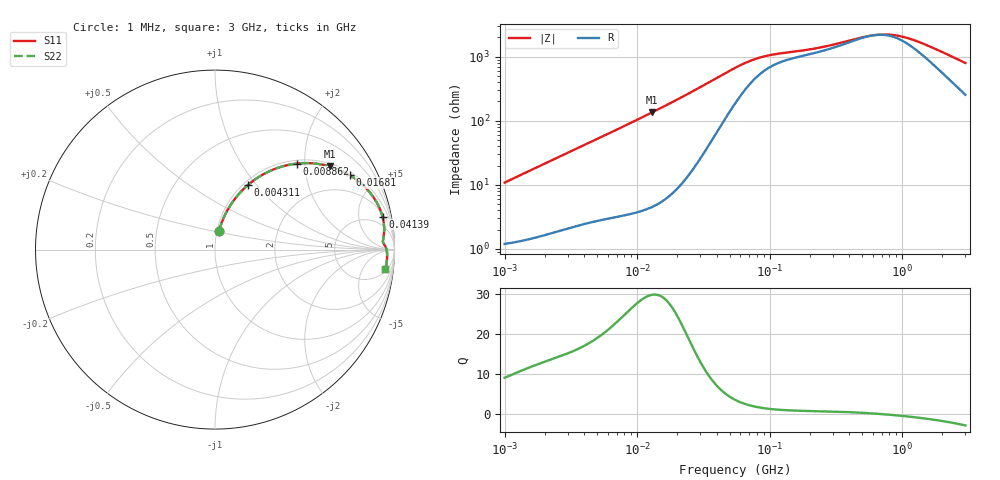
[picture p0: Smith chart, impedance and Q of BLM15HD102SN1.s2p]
! BLM15HD102SN1
# Hz S RI R 50
!Freq.(Hz) S11(Real) S11(Imag) S21(Real) S21(Imag) S12(Real) S12(Imag) S22(Real) S22(Imag)
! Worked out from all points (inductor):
!   401 points, 1 MHz to 3 GHz, reference 50 ohm
!   read as one part in series: L = 1.71 uH near 1.041 MHz
!   highest Q = 29.8 at 12.96 MHz (marker M1), where L = 1.65 uH
!   self-resonance near 622.8 MHz
!   S11 on the Smith chart (normalised r, x): 1 MHz: 1.02, +0.22; 4.311 MHz: 1.05, +0.90; 8.862 MHz: 1.07, +1.83; 16.81 MHz: 1.13, +3.54; 41.39 MHz: 2.49, +9.61; 3 GHz: 6, -15
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1000000  0.0229 0.1041  0.9771 -0.1041  0.9771 -0.1041  0.0229 0.1041
2139570  0.0637 0.2096  0.9363 -0.2096  0.9363 -0.2096  0.0637 0.2096
2888807  0.1003 0.2687  0.8997 -0.2687  0.8997 -0.2687  0.1003 0.2687
3823119  0.1526 0.3309  0.8474 -0.3309  0.8474 -0.3309  0.1526 0.3309
4310966  0.1819 0.3584  0.8181 -0.3584  0.8181 -0.3584  0.1819 0.3584
6058321  0.2914 0.4313  0.7086 -0.4313  0.7086 -0.4313  0.2914 0.4313
8861669  0.4577 0.4794  0.5423 -0.4794  0.5423 -0.4794  0.4577 0.4794
1.29622e7  0.6405 0.4634  0.3595 -0.4634  0.3595 -0.4634  0.6405 0.4634
1.461624e7  0.6939 0.4443  0.3061 -0.4443  0.3061 -0.4443  0.6939 0.4443
1.681455e7  0.7503 0.4155  0.2497 -0.4155  0.2497 -0.4155  0.7503 0.4155
2.559965e7  0.873 0.3055  0.127 -0.3055  0.127 -0.3055  0.873 0.3055
4.138676e7  0.9333 0.1838  0.0667 -0.1838  0.0667 -0.1838  0.9333 0.1838
5.477226e7  0.9422 0.1302  0.0578 -0.1302  0.0578 -0.1302  0.9422 0.1302
7.248696e7  0.9416 0.0918  0.0584 -0.0918  0.0584 -0.0918  0.9416 0.0918
9.216659e7  0.9386 0.0697  0.0614 -0.0697  0.0614 -0.0697  0.9386 0.0697
2.094008e8  0.9381 0.0356  0.0619 -0.0356  0.0619 -0.0356  0.9381 0.0356
5.583748e8  0.9546 0.00455  0.0454 -0.00455  0.0454 -0.00455  0.9546 0.00455
6.685918e8  0.9566 -0.00307  0.0434 0.00307  0.0434 0.00307  0.9566 -0.00307
8.005644e8  0.958 -0.0113  0.042 0.0113  0.042 0.0113  0.958 -0.0113
9.977393e8  0.9589 -0.0224  0.0411 0.0224  0.0411 0.0224  0.9589 -0.0224
1.268618e9  0.9591 -0.036  0.0409 0.036  0.0409 0.036  0.9591 -0.036
3e9  0.949 -0.1088  0.051 0.1088  0.051 0.1088  0.949 -0.1088
